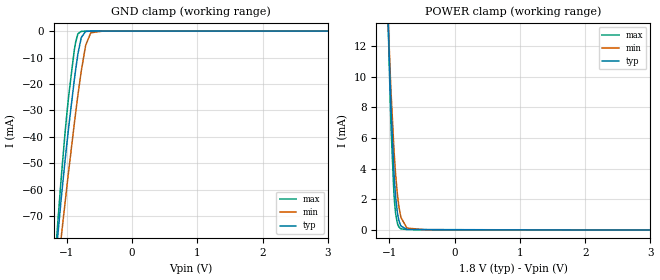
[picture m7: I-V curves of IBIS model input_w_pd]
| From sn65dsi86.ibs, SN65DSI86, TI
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|   Model
[Model]   input_w_pd
Model_type   Input
Vinl = 0.54
Vinh = 1.26
|   typ   min   max
C_comp   1.197pF   1.128pF   1.271pF
[Voltage Range]   1.8   1.65   1.98
[Temperature Range]   27   125   -40
[Power Clamp Reference]   1.8   1.65   1.98
[GND Clamp Reference]   -0   -0   -0
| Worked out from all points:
|   GND clamp passes 1 mA (typ) near -0.74 V on its own axis
|   POWER clamp passes 1 mA (typ) near -0.87 V on its own axis
[GND Clamp]
|   Voltage   I(typ)   I(min)   I(max)
-1.8V     -308mA     -294.7mA   -317.4mA
-1.217V   -100.4mA   -108.5mA   -98.83mA
-1.141V   -77.88mA   -90.3mA    -72.9mA
-1.087V   -63.42mA   -77.99mA   -55.59mA
-968.4mV  -35.53mA   -52.05mA   -23.66mA
-865.8mV  -14.62mA   -30.95mA   -4.205mA
-828mV    -8.224mA   -23.68mA   -969.9uA
-779.4mV  -2.437mA   -15.04mA   -109.5uA
-709.2mV  -141.2uA   -5.191mA   -11.34uA
-633.6mV  -9.437uA   -646.9uA   -6.307uA
-450mV    -3.595uA   -3.858uA   -4.386uA
3.595V    0A         0A         0A
[POWER Clamp]
|   Voltage   I(typ)   I(min)   I(max)
-1.8V     160.6mA    133.1mA    189.1mA
-1.028V   14.82mA    14.62mA    14.83mA
-984.6mV  9.105mA    9.969mA    8.037mA
-973.8mV  7.856mA    8.923mA    6.609mA
-930.6mV  3.802mA    5.313mA    2.391mA
-903.6mV  2.135mA    3.587mA    1.043mA
-876.6mV  1.099mA    2.291mA    416.3uA
-855mV    619.4uA    1.544mA    199.8uA
-828mV    296.1uA    908.6uA    88.11uA
-730.8mV  34.98uA    121.8uA    27.8uA
-450mV    17.99uA    14.3uA     23.71uA
3.595V    0A         0A         0A
